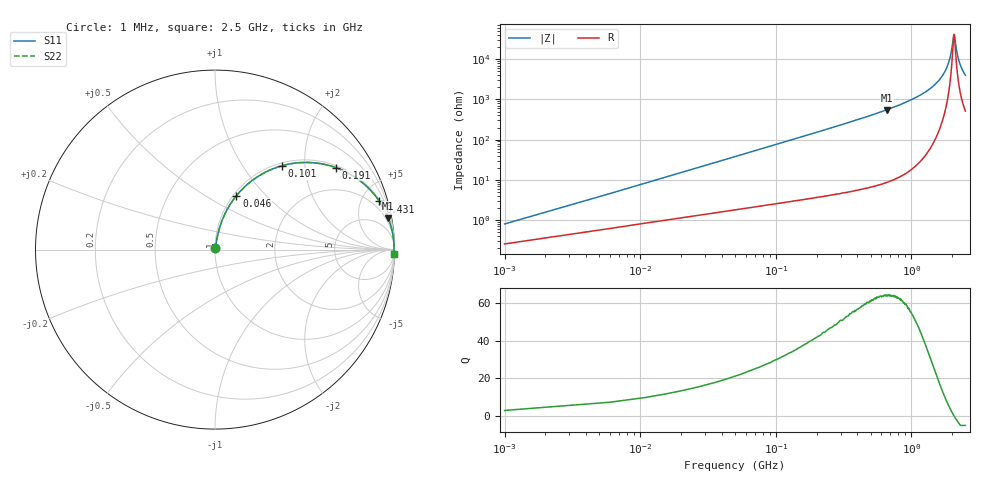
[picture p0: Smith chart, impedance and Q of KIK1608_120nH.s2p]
!version-2
!date-01.2022
!Series
# MHz S RI R 50
!Freq ReS11 ImS11 ReS21 ImS21 ReS12 ImS12 ReS22 ImS22
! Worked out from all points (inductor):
!   501 points, 1 MHz to 2.5 GHz, reference 50 ohm
!   read as one part in series: L = 120 nH near 11 MHz
!   highest Q = 64.1 at 656 MHz (marker M1), where L = 134 nH
!   self-resonance near 2.06 GHz
!   S11 on the Smith chart (normalised r, x): 1 MHz: 1.01, +0.02; 46 MHz: 1.03, +0.69; 101 MHz: 1.05, +1.53; 191 MHz: 1.07, +2.91; 431 MHz: 1.12, +6.79; 2.5 GHz: 11, -80
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1  0.00257 0.0075  0.9974 -0.0075  0.9974 -0.0075  0.00257 0.0075
16  0.0239 0.1166  0.9761 -0.1166  0.9761 -0.1166  0.0239 0.1166
21  0.0351 0.1511  0.9649 -0.1511  0.9649 -0.1511  0.0351 0.1511
31  0.0636 0.2159  0.9364 -0.2159  0.9364 -0.2159  0.0636 0.2159
46  0.1193 0.3005  0.8807 -0.3005  0.8807 -0.3005  0.1193 0.3005
101  0.3725 0.4671  0.6275 -0.4671  0.6275 -0.4671  0.3725 0.4671
191  0.6746 0.4565  0.3254 -0.4565  0.3254 -0.4565  0.6746 0.4565
286  0.8237 0.3711  0.1763 -0.3711  0.1763 -0.3711  0.8237 0.3711
421  0.9125 0.274  0.0875 -0.274  0.0875 -0.274  0.9125 0.274
431  0.9164 0.2683  0.0835 -0.2683  0.0835 -0.2683  0.9164 0.2683
656  0.9655 0.1749  0.0345 -0.1749  0.0345 -0.1749  0.9655 0.1749
836  0.9807 0.1298  0.0193 -0.1298  0.0193 -0.1298  0.9807 0.1298
1255  0.9939 0.066  0.00609 -0.066  0.00609 -0.066  0.9939 0.066
1670  0.9973 0.0272  0.00266 -0.0272  0.00266 -0.0272  0.9973 0.0272
1880  0.9977 0.0119  0.00229 -0.0119  0.00229 -0.0119  0.9977 0.0119
1965  0.9977 0.00625  0.0023 -0.00625  0.0023 -0.00625  0.9977 0.00625
2050  0.9976 0.000838  0.00238 -0.000838  0.00238 -0.000838  0.9976 0.000838
2085  0.9976 -0.00132  0.00244 0.00132  0.00244 0.00132  0.9976 -0.00132
2155  0.9974 -0.00554  0.00258 0.00554  0.00258 0.00554  0.9974 -0.00554
2235  0.9972 -0.0102  0.00279 0.0102  0.00279 0.0102  0.9972 -0.0102
2350  0.9968 -0.0166  0.00317 0.0166  0.00317 0.0166  0.9968 -0.0166
2500  0.9962 -0.0245  0.00379 0.0245  0.00379 0.0245  0.9962 -0.0245
